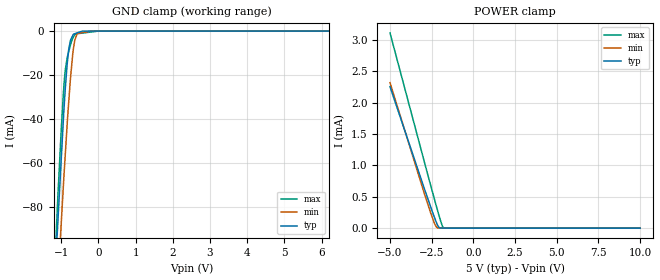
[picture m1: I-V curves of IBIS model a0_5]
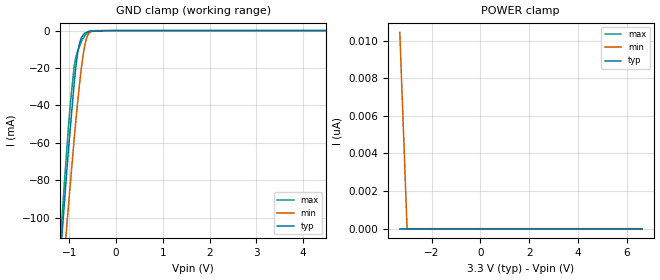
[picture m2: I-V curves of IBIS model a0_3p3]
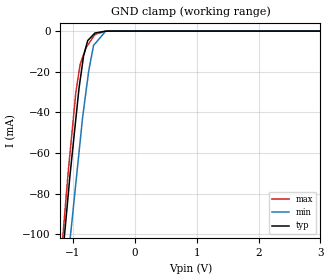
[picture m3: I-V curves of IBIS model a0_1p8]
|Texas Instruments Incorporated
| 8-Channel I2C Switch With Reset
| Marketing part#   Digital Voltage Range   Package-type   #pins
| TCA9548APWR   1.65V-5.5V   TSSOP   24
[IBIS Ver]   4.1
[File name]   tca9548a.ibs
[File Rev]   1.1
[Date]   6/26/2014
[Source]
| Texas Instruments Incorporated.
| Analog-eLab Design Center, HPA
| 12500 TI Blvd
| Dallas, TX -75243
[Notes]   Revision History:
| Rev 1.1: 6/26/2014
| - Add RGE component
| Rev 1.0: 2/18/2013
| - Initial version of the model
| - Model generated from simulations in TISPICE
| - Model matched to SPICE simulation
| - C_comp although listed in numerical order of value are
|   obtained from varying PVT conditions. For PVT conditions for
|   each specific value refer the buffer description under
|   respective [Model]. IBIS model user is responsible for using
|   appropriate C_comp to simulate for Signal Integrity.
[Disclaimer]
| This model is designed as an aid for customers of Texas Instruments.
| TI and its licensors and suppliers make no warranties, either expressed
| or implied, with respect to this  model, including the warranties of
| merchantability or fitness for a particular purpose. The model is
| provided solely on an "as is" basis. The entire risk as to its quality
| and performance is with the customer.
[Copyright]
(C) Copyright 2013 Texas Instruments Incorporated.All rights reserved.
[Component]   TCA9548APWR
[Manufacturer]   TI
[Package]   |24-TSSOP
|   typ   min   max
R_pkg   0.08565   0.08015   0.08885
L_pkg   3.98044nH   3.45983nH   4.53722nH
C_pkg   0.60633pF   0.50443pF   0.68004pF
[Pin]  signal_name   model_name   R_pin   L_pin   C_pin
1   A0   A0   0.08015   4.53722nH  0.68004pF
2   A1   A0   0.08546   4.17243nH  0.66443pF
3   _RESET   A0   0.08885   3.78775nH  0.56415pF
4   SD0   NC   0.08724   3.46324nH  0.50426pF
5   SC0   NC   0.08235   3.22931nH  0.49221pF
6   SD1   NC   0.07789   3.08150nH  0.45958pF
7   SC1   NC   0.07794   3.08257nH  0.46003pF
8   SD2   NC   0.08249   3.23564nH  0.49286pF
9   SC2   NC   0.08746   3.47313nH  0.50532pF
10   SD3   NC   0.08912   3.80197nH  0.56781pF
11   SC3   NC   0.08216   4.11724nH  0.65915pF
12   GND   GND   0.07890   4.52785nH  0.67433pF
13   SD4   NC   0.07997   4.54202nH  0.67661pF
14   SC4   NC   0.08253   4.12145nH  0.66060pF
15   SD5   NC   0.08932   3.80465nH  0.56826pF
16   SC5   NC   0.08762   3.47654nH  0.50517pF
17   SD6   NC   0.08259   3.23769nH  0.49271pF
18   SC6   NC   0.07798   3.08419nH  0.45984pF
19   SD7   NC   0.07785   3.07907nH  0.45994pF
20   SC7   NC   0.08225   3.22733nH  0.49238pF
21   A2   A0   0.08708   3.45983nH  0.50443pF
22   SCL   SCL   0.08865   3.78507nH  0.56384pF
23   SDA   SDA   0.08371   4.14035nH  0.66107pF
24   VCC   POWER   0.08002   4.54204nH  0.67905pF
[Component]   TCA9548ARGE
[Manufacturer]   TI
[Package]   |24-VQFN
|   typ   min   max
R_pkg   0.1156   0.0998   0.1325
L_pkg   1.7061n   1.4583n   1.9744n
C_pkg   0.2181p   0.2059p   0.2270p
[Pin]  signal_name   model_name   R_pin   L_pin   C_pin
1   SD0   NC   0.13201  1.97025n  0.22256p
2   SC0   NC   0.11651  1.72122n  0.22675p
3   SD1   NC   0.10980  1.61632n  0.21843p
4   SC1   NC   0.10987  1.61732n  0.21851p
5   SD2   NC   0.11669  1.72402n  0.22698p
6   SC2   NC   0.13227  1.97438n  0.22297p
7   SD3   NC   0.12786  1.90445n  0.21954p
8   SC3   NC   0.10515  1.54281n  0.21367p
9   GND   GND   0.09980  1.45832n  0.20588p
10   SD4   NC   0.10120  1.47832n  0.20758p
11   SC4   NC   0.10559  1.54592n  0.21397p
12   SD5   NC   0.12813  1.90278n  0.21928p
13   SC5   NC   0.13246  1.96945n  0.22295p
14   SD6   NC   0.11683  1.71761n  0.22686p
15   SC6   NC   0.10992  1.60892n  0.21825p
16   SD7   NC   0.10976  1.60642n  0.21807p
17   SC7   NC   0.11638  1.71061n  0.22630p
18   A2   A0   0.13181  1.95924n  0.22210p
19   SCL   SCL   0.12725  1.88905n  0.21563p
20   SDA   SDA   0.10691  1.56602n  0.21488p
21   VCC   POWER   0.10123  1.47872n  0.20986p
22   A0   A0   0.10134  1.48192n  0.21032p
23   A1   A0   0.10900  1.60271n  0.21730p
24   _RESET   A0   0.12751  1.89894n  0.21563p
|   Model Selectors
[Model Selector] A0
a0_5   5.0V digital input
a0_3p3  3.3V digital input
a0_1p8  1.8V digital input
[Model Selector] SCL
scl_5   5.0V digital input
scl_3p3  3.3V digital input
scl_1p8  1.8V digital input
[Model Selector] SDA
sda_5   5.0V digital I/O Open_Drain
sda_3p3  3.3V digital I/O Open_Drain
sda_1p8  1.8V digital I/O Open_Drain
| Models and submodels in the file (9): a0_5 (Input), a0_3p3 (Input), a0_1p8 (Input), scl_5 (Input), scl_3p3 (Input), scl_1p8 (Input), sda_5 (I/O_open_drain), sda_3p3 (I/O_open_drain), sda_1p8 (I/O_open_drain)
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|   a0_5 Model
[Model]   a0_5
Model_type   Input
Vinl = 1.5
Vinh = 3.5
|   typ   min   max
|   (nom PVT)   (fast PVT)   (slow PVT)
 C_comp   1.359e-12   1.280e-12   1.465e-12
[Model spec]
|subparameter
Vinl   1.5   1.35   1.65
Vinh   3.5   3.15   3.85
|Where nom  PVT is Nominal Process, 5V, 27C
|   Fast PVT is Strong Process,  5.5V, -40C
|   Slow PVT is Weak Process,   4.5V, 125C
[Voltage Range]   5   4.5   5.5
|Junction Temperature
[Temperature Range]   27   125   -40
[Power Clamp Reference]   5   4.5   5.5
[GND Clamp Reference]   0   0   0
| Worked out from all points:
|   GND clamp passes 1 mA (typ) near -0.60 V on its own axis
[GND Clamp]
|   Voltage   I(typ)   I(min)   I(max)
-5V       -1.628A    -1.544A    -1.73A
-1.14V    -101.9mA   -130.3mA   -93.4mA
-1.095V   -87.6mA    -115.6mA   -76.26mA
-1.001V   -58.26mA   -87.41mA   -44.81mA
-907.5mV  -30.13mA   -60.17mA   -20.44mA
-845mV    -15.62mA   -43.39mA   -12.61mA
-800mV    -8.434mA   -32.44mA   -9.323mA
-756mV    -4.582mA   -22.18mA   -6.585mA
-670mV    -1.391mA   -7.626mA   -2.629mA
-571.5mV  -815.3uA   -1.062mA   -1.195mA
-202.5mV  -8.304uA   -179.7nA   -423.5uA
10V       0A         0A         0A
[POWER Clamp]
|   Voltage   I(typ)   I(min)   I(max)
-5V       2.258mA    2.32mA     3.114mA
-2.934V   625.5uA    546.7uA    1.051mA
-2.542V   326uA      227.7uA    664.8uA
-2.317V   160.2uA    66.42uA    444.9uA
-2.219V   91.38uA    18.22uA    349.3uA
-2.09V    19.61uA    2.399uA    227.7uA
-2.015V   2.464uA    2.149uA    160.3uA
-1.859V   1.864uA    1.629uA    33.39uA
-1.793V   1.61uA     1.409uA    5.051uA
10V       0A         0A         0A
|   a0_3p3 Model
[Model]   a0_3p3
Model_type   Input
Vinl = 0.99
Vinh = 2.31
|   typ   min   max
|   (nom PVT)   (fast PVT)   (slow PVT)
C_comp   1.365e-12   1.304e-12   1.465e-12
[Model spec]
|subparameter
Vinl   0.99   0.9   1.08
Vinh   2.31   2.1   2.52
|Where nom  PVT is Nominal Process, 3.3V, 27C
|   Fast PVT is Strong Process,  3.6V, -40C
|   Slow PVT is Weak Process,   3V, 125C
[Voltage Range]   3.3   3   3.6
|Junction Temperature
[Temperature Range]   27   125   -40
[Power Clamp Reference]   3.3   3   3.6
[GND Clamp Reference]   0   0   0
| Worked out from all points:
|   GND clamp passes 1 mA (typ) near -0.64 V on its own axis
[GND Clamp]
|   Voltage   I(typ)   I(min)   I(max)
-3.3V     -936mA     -899.3mA   -992.4mA
-1.208V   -125mA     -151.4mA   -118.4mA
-1.112V   -93.32mA   -121.1mA   -82.62mA
-1.047V   -71.63mA   -101mA     -60.03mA
-982.8mV  -52.28mA   -82.25mA   -39.24mA
-896.4mV  -27.28mA   -57.07mA   -18.52mA
-821.7mV  -11.49mA   -37.68mA   -10.75mA
-785.4mV  -6.806mA   -28.67mA   -8.483mA
-693mV    -1.901mA   -10.72mA   -3.597mA
-590.7mV  -406.7uA   -1.646mA   -945.6uA
-285mV    -142.3uA   -1.35uA    -11.68uA
6.6V      0A         0A         0A
[POWER Clamp]
|   Voltage   I(typ)   I(min)   I(max)
-3.3V     0A         10.43nA    0A
-3.298V   0A         10.42nA    0A
-3V       0A         0A         0A
6.6V      0A         0A         0A
|   a0_1p8 Model
[Model]   a0_1p8
Model_type   Input
Vinl = 0.54
Vinh = 1.26
|   typ   min   max
|   (nom PVT)   (fast PVT)   (slow PVT)
C_comp   1.391e-12   1.340e-12   1.465e-12
[Model spec]
|subparameter
Vinl   0.54   0.513   0.567
Vinh   1.26   1.197   1.323
| Where nom  PVT is Nominal Process, 1.8V, 27C
|   Fast PVT is Strong Process,  1.89V, -40C
|   Slow PVT is Weak Process,   1.71V, 125C
[Voltage Range]   1.8   1.71   1.89
[Temperature Range]   27   125   -40
[Power Clamp Reference]   1.8   1.71   1.89
[GND Clamp Reference]   0   0   0
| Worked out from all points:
|   GND clamp passes 1 mA (typ) near -0.64 V on its own axis
[GND Clamp]
|   Voltage   I(typ)   I(min)   I(max)
-1.8V     -342.1mA   -350.9mA   -353.9mA
-1.197V   -121.2mA   -147.9mA   -114.1mA
-1.074V   -80.2mA    -111.2mA   -68.91mA
-1.046V   -70.99mA   -103mA     -60.15mA
-948.8mV  -42.45mA   -74.2mA    -29.68mA
-882.6mV  -24.36mA   -54.56mA   -16.48mA
-826.2mV  -12.22mA   -38.81mA   -11.58mA
-743.9mV  -4.171mA   -19.68mA   -6.239mA
-665.2mV  -1.659mA   -7.048mA   -2.698mA
-642.6mV  -937.4uA   -6.242mA   -1.681mA
-456.6mV  -33.92uA   -70uA      -36.22uA
3.6V      0A         0A         0A
[POWER Clamp]
|   Voltage   I(typ)   I(min)   I(max)
-1.8V     0A         0A         0A
-1.799V   0A         0A         0A
3.6V      0A         0A         0A
